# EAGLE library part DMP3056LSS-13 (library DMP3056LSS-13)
MOSFET P Channel 30V 7.1A 2.1V @ 250uA 45m @ 6A,10V SOP-8_150mil RoHS Source: Datasheet
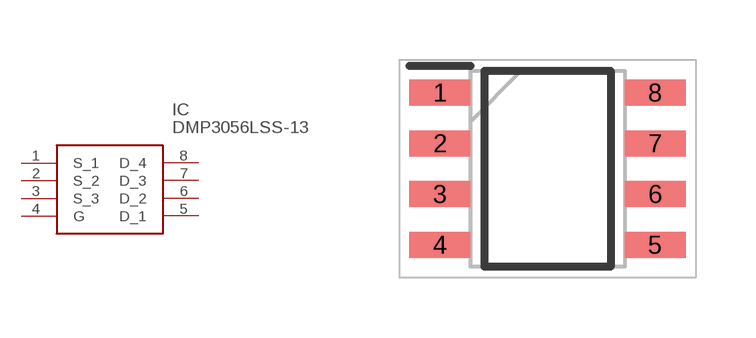
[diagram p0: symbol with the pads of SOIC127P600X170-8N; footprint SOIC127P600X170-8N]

Designator prefix IC

## DMP3056LSS-13 (Description: MOSFET P Channel 30V 7.1A 2.1V @ 250uA 45m @ 6A,10V SOP-8_150mil RoHS; Height: 1.7mm; Manufacturer_Name: Diodes Incorporated; Manufacturer_Part_Number: DMP3056LSS-13; Mouser_Part_Number: 621-DMP3056LSS-13; Mouser_Price-Stock: https://www.mouser.co.uk/ProductDetail/Diodes-Incorporated/DMP3056LSS-13?qs=oUsD4qhOtFyEnPLZKitYRA%3D%3D)  [SOIC127P600X170-8N]
1  S_1
2  S_2
3  S_3
4  G
5  D_1
6  D_2
7  D_3
8  D_4

## Footprint SOIC127P600X170-8N (pad centres in mm)
DMP3056LSS-13
smd 1.525 x 0.65: 1 -2.688,1.905; 2 -2.688,0.635; 3 -2.688,-0.635; 4 -2.688,-1.905; 5 2.688,-1.905; 6 2.688,-0.635; 7 2.688,0.635; 8 2.688,1.905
